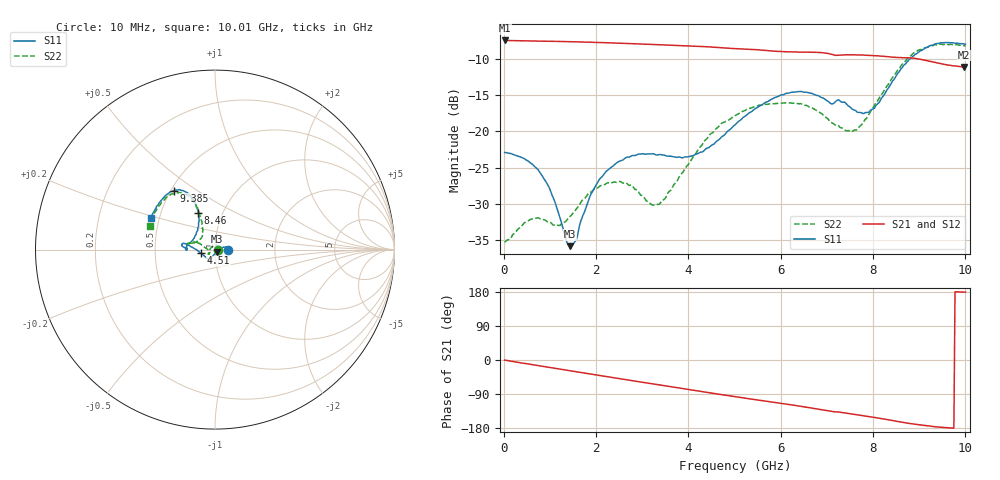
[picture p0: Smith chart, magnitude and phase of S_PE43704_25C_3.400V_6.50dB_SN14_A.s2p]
! Device ID: PE43704
! Dir: z:\PE43704\PE43704_Char_1_20130516\PE43704\AMB\3p400V\6p50dB
! Serial: 14
! Insertion: A
! Impedance: 50 ohm
! Temp: Amb
! VDD: 3.400V
! Attenuation Step: 6.50dB
! IDD: 1.140341e-01mA
#  Hz  S  RI  R  50
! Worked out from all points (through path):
!   401 points, 10 MHz to 10.01 GHz, reference 50 ohm
!   highest |S21| = -7.50 dB at 10 MHz (marker M1); lowest = -11.2 dB at 9.985 GHz (marker M2)
!   group delay of S21, straight-line fit = 51.7 ps
!   lowest |S11| = -35.8 dB at 1.435 GHz (marker M3), VSWR 1.03, Z = 51.2 - j1.15 ohm
!   |S11| at or under -10 dB: start of sweep to 8.815 GHz
!   |S22| runs from -35.3 to -8.0 dB; largest |S21 - S12| = 0.0034
!   S11 on the Smith chart (normalised r, x): 10 MHz: 1.15, +0.00; 4.51 GHz: 0.86, -0.04; 8.46 GHz: 0.77, +0.33; 9.385 GHz: 0.52, +0.41; 10.01 GHz: 0.45, +0.19
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1e7  0.0714 9.94e-05  0.4218 -0.00165  0.4221 -0.00164  0.0172 0.000472
7.85e8  0.0496 0.0142  0.4017 -0.1128  0.4017 -0.1126  0.00248 0.0248
1.16e9  0.0285 0.00305  0.3822 -0.1626  0.3822 -0.1624  -0.0139 0.0178
1.435e9  0.0117 -0.0112  0.3636 -0.1969  0.3636 -0.1967  -0.0253 0.00641
1.685e9  -0.00188 -0.0251  0.344 -0.2264  0.344 -0.2261  -0.0327 -0.0059
1.935e9  -0.0122 -0.0375  0.3219 -0.2533  0.3219 -0.2532  -0.0361 -0.0161
2.26e9  -0.0208 -0.0503  0.2899 -0.285  0.29 -0.2848  -0.037 -0.0241
2.685e9  -0.0274 -0.0606  0.2437 -0.3198  0.244 -0.3202  -0.035 -0.0252
3.36e9  -0.0347 -0.0597  0.1632 -0.359  0.1637 -0.3588  -0.0302 -0.00847
4.035e9  -0.0543 -0.0398  0.0777 -0.3782  0.0782 -0.3783  -0.0598 0.0144
4.51e9  -0.0777 -0.0211  0.0164 -0.3794  0.0169 -0.3797  -0.0906 0.0349
5.01e9  -0.1106 0.00355  -0.043 -0.3682  -0.0427 -0.3685  -0.1228 0.0363
5.96e9  -0.1713 0.0348  -0.1422 -0.3248  -0.1411 -0.3252  -0.1517 0.0357
6.685e9  -0.1813 0.0179  -0.2109 -0.2792  -0.2109 -0.2788  -0.1399 0.037
7.585e9  -0.1335 0.0431  -0.269 -0.2014  -0.2686 -0.2013  -0.0742 0.0691
7.96e9  -0.1034 0.0945  -0.2884 -0.1655  -0.2884 -0.1661  -0.0697 0.1197
8.36e9  -0.0898 0.1824  -0.3019 -0.1206  -0.302 -0.122  -0.0849 0.1991
8.46e9  -0.0931 0.2067  -0.3041 -0.1081  -0.3043 -0.1096  -0.0948 0.221
8.91e9  -0.1419 0.3056  -0.3125 -0.0593  -0.3109 -0.0591  -0.1644 0.3079
9.385e9  -0.2301 0.3284  -0.2955 -0.0183  -0.2965 -0.0175  -0.2531 0.3013
9.985e9  -0.3514 0.1859  -0.277 0.00378  -0.278 0.0053  -0.3604 0.142
1.001e10  -0.357 0.1759  -0.2778 0.00426  -0.2794 0.00467  -0.3638 0.1332
